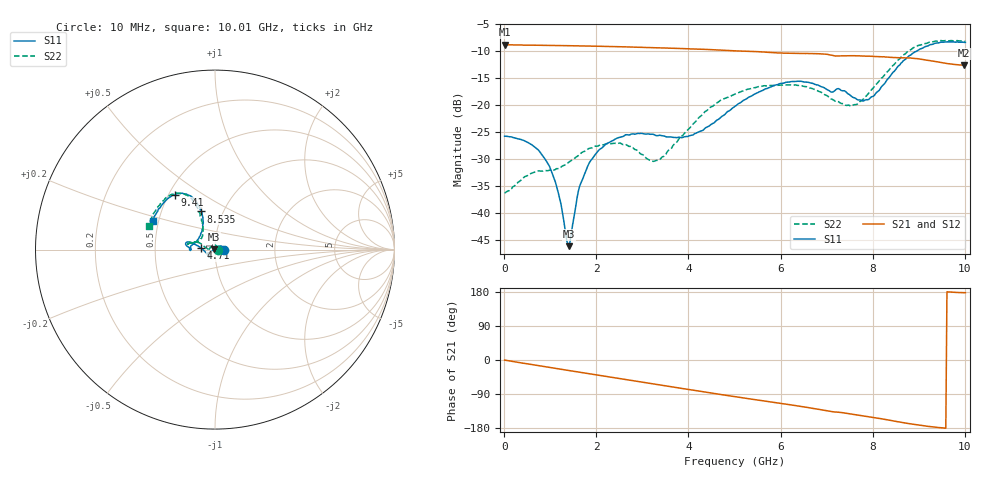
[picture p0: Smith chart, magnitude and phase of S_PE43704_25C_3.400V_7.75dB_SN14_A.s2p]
! Device ID: PE43704
! Dir: z:\PE43704\PE43704_Char_1_20130516\PE43704\AMB\3p400V\7p75dB
! Serial: 14
! Insertion: A
! Impedance: 50 ohm
! Temp: Amb
! VDD: 3.400V
! Attenuation Step: 7.75dB
! IDD: 1.139512e-01mA
#  Hz  S  RI  R  50
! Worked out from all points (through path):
!   401 points, 10 MHz to 10.01 GHz, reference 50 ohm
!   highest |S21| = -8.78 dB at 10 MHz (marker M1); lowest = -12.6 dB at 9.985 GHz (marker M2)
!   group delay of S21, straight-line fit = 52 ps
!   lowest |S11| = -46.1 dB at 1.41 GHz (marker M3), VSWR 1.01, Z = 49.6 + j0.269 ohm
!   |S11| at or under -10 dB: start of sweep to 8.944 GHz
!   |S22| runs from -36.3 to -8.0 dB; largest |S21 - S12| = 0.0027
!   S11 on the Smith chart (normalised r, x): 10 MHz: 1.11, +0.00; 4.71 GHz: 0.86, +0.01; 8.535 GHz: 0.79, +0.35; 9.41 GHz: 0.54, +0.39; 10.01 GHz: 0.46, +0.17
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1e7  0.0516 0.000212  0.3639 -0.00139  0.364 -0.00129  0.0153 0.000425
5.6e8  0.0402 0.018  0.3539 -0.0702  0.354 -0.0702  0.00708 0.022
9.35e8  0.0229 0.0186  0.3404 -0.1142  0.3404 -0.114  -0.00708 0.0237
1.135e9  0.0113 0.0139  0.3311 -0.1373  0.3312 -0.137  -0.0167 0.0197
1.36e9  -0.00162 0.00528  0.3185 -0.1615  0.3184 -0.1613  -0.0264 0.0115
1.41e9  -0.00412 0.00272  0.3153 -0.1667  0.3154 -0.1666  -0.0283 0.00934
1.685e9  -0.0172 -0.00989  0.297 -0.1947  0.2972 -0.1945  -0.0363 -0.00319
1.885e9  -0.0245 -0.0189  0.282 -0.2134  0.2821 -0.2133  -0.0383 -0.0117
2.235e9  -0.0309 -0.0316  0.2529 -0.2435  0.2531 -0.2433  -0.0393 -0.0202
3.36e9  -0.0355 -0.0389  0.1413 -0.3101  0.1416 -0.3098  -0.0305 -0.00567
4.035e9  -0.0488 -0.0189  0.067 -0.3264  0.0674 -0.3264  -0.0595 0.0174
4.71e9  -0.0774 0.00772  -0.00728 -0.3239  -0.0071 -0.324  -0.1043 0.0429
5.01e9  -0.0954 0.0203  -0.0374 -0.3175  -0.0371 -0.3177  -0.1209 0.0388
5.935e9  -0.1495 0.0425  -0.1215 -0.2805  -0.1206 -0.2813  -0.1488 0.0371
6.685e9  -0.1587 0.0213  -0.183 -0.2392  -0.1831 -0.2395  -0.1382 0.036
7.585e9  -0.1105 0.0403  -0.2322 -0.1706  -0.2318 -0.1704  -0.0734 0.0693
7.935e9  -0.0801 0.0837  -0.2476 -0.1416  -0.2476 -0.1421  -0.0676 0.1156
8.36e9  -0.0672 0.169  -0.2596 -0.101  -0.2594 -0.1019  -0.0833 0.1972
8.535e9  -0.0776 0.2129  -0.2639 -0.0823  -0.2635 -0.0843  -0.1025 0.2379
9.41e9  -0.2215 0.3057  -0.2518 -0.00847  -0.2517 -0.00835  -0.2585 0.2958
9.985e9  -0.342 0.1709  -0.2344 0.0097  -0.2352 0.0102  -0.3647 0.1418
1.001e10  -0.3474 0.1604  -0.2348 0.00997  -0.2363 0.00999  -0.3687 0.1332
